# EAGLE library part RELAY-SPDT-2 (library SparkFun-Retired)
SPDT Relay w/ Two Common Terminals SPDT relay (COM-00100)
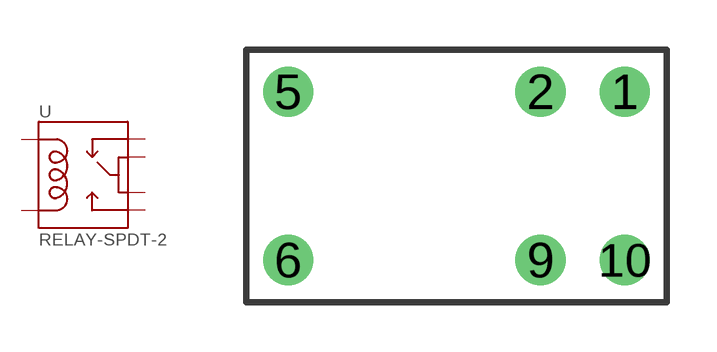
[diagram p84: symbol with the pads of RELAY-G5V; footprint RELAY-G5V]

Designator prefix -

## RELAY-SPDT-2-G5V (SF_SKU: COM-00524)  [RELAY-G5V]
1  1
2  2
5  5
6  6
9  9
10  10

## Footprint RELAY-G5V (pad centres in mm)
G5Q SPDT Relay (SparkFun SKU: COM-00100). Footprint should also work with SPST-NO relay.
drill 1.016: 1 5.08,2.54; 2 2.54,2.54; 5 -5.08,2.54; 6 -5.08,-2.54; 9 2.54,-2.54; 10 5.08,-2.54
